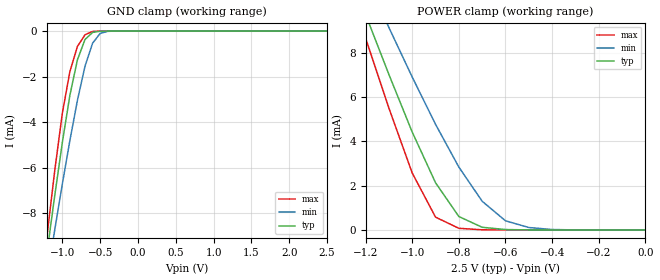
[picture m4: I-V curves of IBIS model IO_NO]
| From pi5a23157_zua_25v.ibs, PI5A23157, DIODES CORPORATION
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[Model]   IO_NO
Model_type   Terminator
C_comp   2.989pF   2.956pF   3.111pF
[Voltage Range]   2.5   2.3   2.7
[Temperature Range]   25   -40   125
[GND Clamp Reference]   0   0   0
[POWER Clamp Reference]   2.5   2.3   2.7
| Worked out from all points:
|   GND clamp passes 1 mA (typ) near -0.77 V on its own axis
|   POWER clamp passes 1 mA (typ) near -0.83 V on its own axis
[GND_Clamp]
-2.5V     -1.685A    -2.018A    -1.463A
-1.2V     -9.674mA   -10.81mA   -8.944mA
-1.1V     -7.224mA   -8.733mA   -6.127mA
-1V       -4.897mA   -6.727mA   -3.616mA
-900mV    -2.821mA   -4.809mA   -1.777mA
-800mV    -1.257mA   -3.037mA   -673.9uA
-700mV    -367.7uA   -1.543mA   -161.9uA
-600mV    -59.25uA   -533uA     -14.42uA
-500mV    -5.324uA   -102.4uA   -563.2nA
-400mV    -316nA     -10.83uA   -13.24nA
2.5V      377.7pA    228.5nA    251.5pA
[Power_Clamp]
-2.5V     36.63mA    31.09mA    40.56mA
-1.3V     12.45mA    13.71mA    11.79mA
-1.2V     9.728mA    11.42mA    8.659mA
-1.1V     7.02mA     9.139mA    5.502mA
-1V       4.42mA     6.903mA    2.574mA
-900mV    2.132mA    4.769mA    579.9uA
-800mV    606.9uA    2.838mA    75.2uA
-700mV    121.6uA    1.296mA    7.847uA
-600mV    18.95uA    412.9uA    573.1nA
-500mV    1.921uA    111uA      23.52nA
-400mV    132.9nA    20.24uA    1.549nA
0V        377.6pA    3.593nA    399.6pA
